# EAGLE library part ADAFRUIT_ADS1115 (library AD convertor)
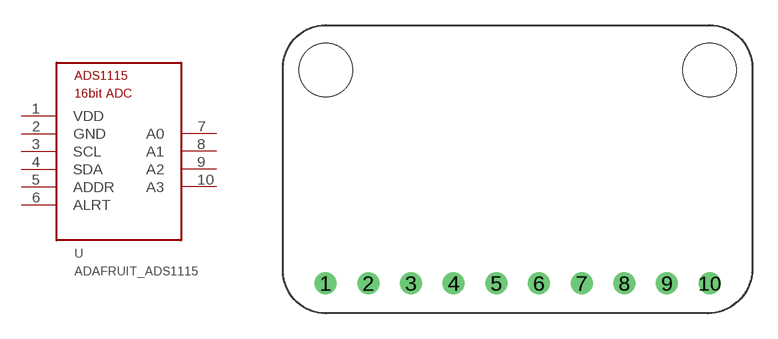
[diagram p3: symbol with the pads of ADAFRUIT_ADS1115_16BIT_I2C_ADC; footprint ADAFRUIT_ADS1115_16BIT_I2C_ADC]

Designator prefix U

## ADAFRUIT_ADS1115  [ADAFRUIT_ADS1115_16BIT_I2C_ADC]
1  VDD
2  GND
3  SCL
4  SDA
5  ADDR
6  ALRT
7  A0
8  A1
9  A2
10  A3

## Footprint ADAFRUIT_ADS1115_16BIT_I2C_ADC (pad centres in mm)
ADS1115 16-Bit ADC - 4 Channel with Programmable Gain Amplifier Maker: adafruit Store: スイッチサイエンス
drill 0.8: 1 2.54,1.778; 2 5.08,1.778; 3 7.62,1.778; 4 10.16,1.778; 5 12.7,1.778; 6 15.24,1.778; 7 17.78,1.778; 8 20.32,1.778; 9 22.86,1.778; 10 25.4,1.778
hole 3.2 at 2.54,14.478
hole 3.2 at 25.4,14.478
